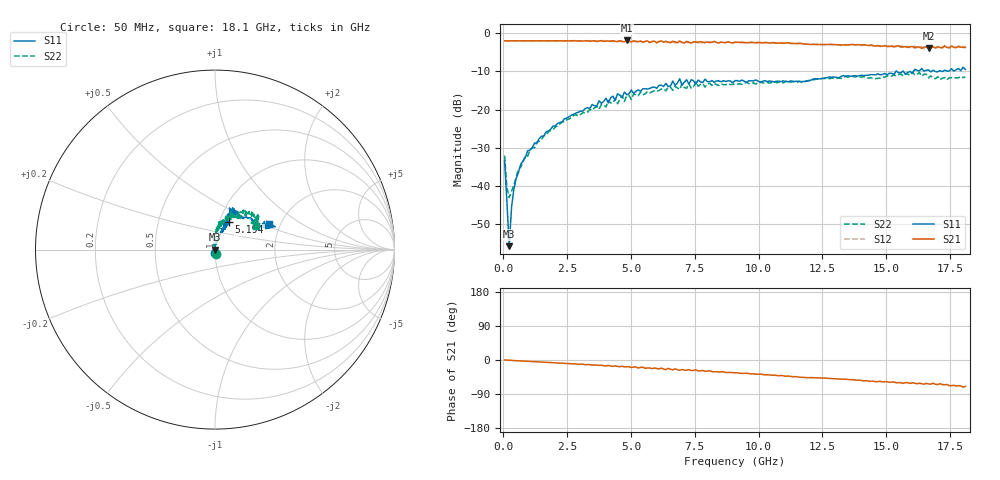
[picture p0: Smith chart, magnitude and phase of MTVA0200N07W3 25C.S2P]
! Network Analyzer HP8720D.06.14 Serial No. US36140669
!  7 Jul 2005  07:22:15
! Frequency  S11  S21  S12  S22
# HZ  S  DB R 50
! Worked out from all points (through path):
!   201 points, 50 MHz to 18.1 GHz, reference 50 ohm
!   highest |S21| = -1.86 dB at 4.833 GHz (marker M1); lowest = -3.9 dB at 16.66 GHz (marker M2)
!   group delay of S21, straight-line fit = 10.7 ps
!   lowest |S11| = -55.9 dB at 230.5 MHz (marker M3), VSWR 1.00, Z = 49.8 + j0.00903 ohm
!   |S11| at or under -10 dB: start of sweep to 15.38 GHz; 15.42 GHz to 15.64 GHz (220.7 MHz wide, 1.42 % of centre); 15.68 GHz to 16.06 GHz (389.2 MHz wide, 2.45 % of centre)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
!   |S22| runs from -43.1 to -10.2 dB; largest |S21 - S12| = 0.046
!   S11 on the Smith chart (normalised r, x): 50 MHz: 1.00, -0.04; 5.194 GHz: 1.11, +0.35; 18.1 GHz: 1.75, +0.57
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5e7  -33.56 -87.2  -1.94 0.1  -1.94 0.2  -32.12 -81.9
1.4025e8  -44.20 -103.6  -1.98 -0.4  -1.97 -0.4  -40.53 -134.8
2.305e8  -55.90 176.8  -1.95 -0.7  -1.95 -0.7  -43.12 -174.7
3.2075e8  -45.76 109.6  -1.94 -0.9  -1.96 -1.0  -41.57 148.1
4.11e8  -41.03 97.5  -1.96 -1.5  -1.95 -1.5  -39.79 135.0
5.915e8  -36.58 91.3  -1.96 -1.9  -1.97 -2.0  -35.59 116.8
9.525e8  -30.85 82.7  -1.95 -3.4  -1.94 -3.3  -32.29 104.4
1.76475e9  -25.65 78.5  -1.93 -6.4  -1.95 -6.6  -25.90 91.4
3.1185e9  -20.39 70.5  -2.02 -11.1  -2.04 -11.6  -20.82 87.8
4.83325e9  -16.13 71.2  -1.86 -17.9  -2.10 -18.7  -16.41 73.4
5.19425e9  -15.24 62.7  -2.17 -18.3  -2.00 -18.6  -16.22 81.8
6.09675e9  -13.70 64.6  -2.17 -23.4  -2.05 -23.0  -15.01 71.2
6.7285e9  -13.70 70.4  -2.22 -23.3  -2.53 -24.3  -13.90 64.4
6.909e9  -11.92 67.0  -2.03 -27.0  -2.15 -24.9  -14.72 64.8
6.99925e9  -13.59 66.7  -2.31 -25.1  -2.49 -27.5  -13.25 64.8
7.17975e9  -12.17 70.9  -2.08 -26.9  -2.40 -25.3  -14.44 60.5
7.54075e9  -13.36 62.7  -2.30 -25.9  -2.14 -29.1  -12.79 67.7
9.075e9  -12.43 62.1  -2.34 -33.6  -2.31 -33.7  -13.27 57.7
1.21435e10  -11.97 46.4  -2.88 -46.5  -2.82 -46.6  -12.20 56.9
1.512175e10  -10.44 24.6  -3.45 -59.0  -3.18 -58.5  -11.22 47.9
1.6656e10  -9.58 24.3  -3.95 -63.3  -3.73 -61.0  -11.69 32.2
1.81e10  -9.48 25.4  -3.62 -69.6  -3.90 -69.6  -11.50 29.9
